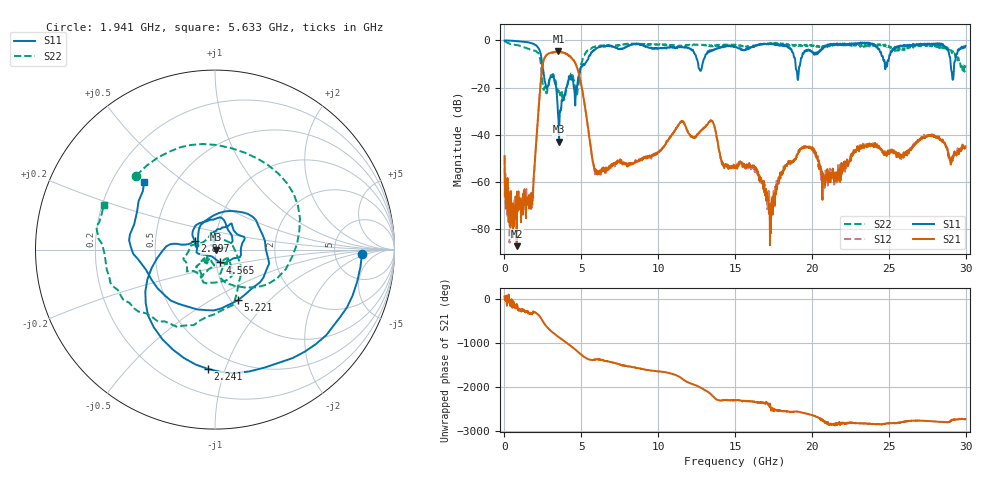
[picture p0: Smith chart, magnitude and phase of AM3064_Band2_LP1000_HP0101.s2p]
# Hz S DB R 50.0
!freq dBS11 angS11 dBS21 angS21 dBS12 angS12 dBS22 angS22
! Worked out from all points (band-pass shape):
!   1600 points, 10 MHz to 29.98 GHz, reference 50 ohm
!   highest |S21| = -4.70 dB at 3.515 GHz (marker M1); lowest = -87.1 dB at 797.2 MHz (marker M2)
!   |S21| within 3 dB of the highest: 2.591 GHz to 4.402 GHz (1.81 GHz wide, 51.8 % of centre)
!   lowest |S11| = -42.9 dB at 3.553 GHz (marker M3), VSWR 1.01, Z = 50.7 - j0.00343 ohm
!   |S11| at or under -10 dB: 2.452 GHz to 5.24 GHz (2.788 GHz wide, 72.5 % of centre); 12.6 GHz to 12.88 GHz (281.6 MHz wide, 2.21 % of centre); 18.93 GHz to 19.23 GHz (301 MHz wide, 1.58 % of centre)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
!   |S22| runs from -25.2 to -0.2 dB; largest |S21 - S12| = 0.012
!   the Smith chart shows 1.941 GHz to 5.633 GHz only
!   S11 on the Smith chart (normalised r, x): 1.941 GHz: 9.88, -1.31; 2.241 GHz: 0.37, -0.87; 2.897 GHz: 0.79, +0.08; 4.565 GHz: 1.05, -0.15; 5.221 GHz: 1.07, -0.67; 5.633 GHz: 0.34, +0.36
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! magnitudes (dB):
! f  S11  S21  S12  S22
! 10 MHz  0.0  -49.0  -49.5  -0.2
! 328.6 MHz  -0.2  -65.0  -85.7  -1.4
! 797.2 MHz  -0.3  -87.1  -71.6  -2.0
! 1.941 GHz  -1.7  -55.2  -54.3  -4.4
! 2.241 GHz  -3.5  -27.4  -27.3  -5.9
! 2.897 GHz  -18.2  -5.5  -5.5  -17.1
! 3.515 GHz  -33.5  -4.7  -4.8  -21.9
! 3.553 GHz  -42.9  -5.0  -4.9  -21.0
! 4.565 GHz  -22.3  -9.1  -9.0  -18.4
! 5.015 GHz  -11.2  -19.4  -19.4  -9.7
! 5.221 GHz  -10.2  -27.2  -27.2  -5.8
! 5.633 GHz  -5.3  -46.3  -46.3  -3.5
! 6.045 GHz  -3.2  -56.2  -56.8  -2.5
! 10 GHz  -3.4  -47.3  -47.7  -1.8
! 13.43 GHz  -4.6  -33.9  -33.9  -2.5
! 15 GHz  -2.5  -53.8  -53.8  -1.8
! 16.3 GHz  -2.1  -54.6  -54.2  -2.1
! 17.31 GHz  -1.6  -69.0  -73.8  -1.3
! 19.99 GHz  -4.5  -46.2  -45.7  -1.9
! 20.93 GHz  -2.3  -56.9  -58.5  -2.1
! 25 GHz  -8.1  -46.9  -47.0  -2.3
! 29.98 GHz  -2.3  -44.8  -46.1  -10.6
